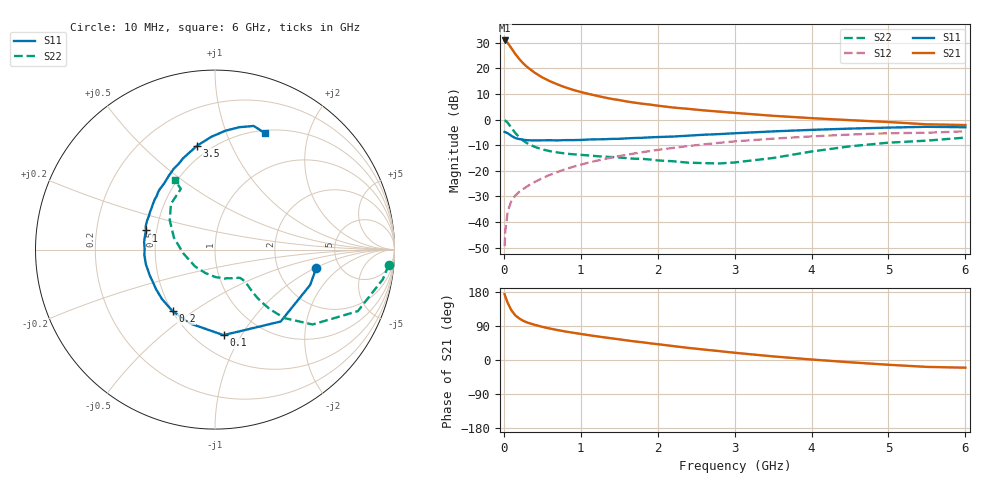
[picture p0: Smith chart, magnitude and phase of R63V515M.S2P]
! SIEMENS Small Signal Semiconductors
! BFR193
! Si NPN RF Bipolar Junction Transistor in SOT23
! VCE = 3.5 V  IC = 15 mA
! Common Emitter S-Parameters:  May  1996
# GHz  S  MA  R  50
!  f  S11  S21  S12  S22
! GHz  MAG  ANG  MAG  ANG  MAG  ANG  MAG  ANG
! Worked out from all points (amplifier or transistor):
!   36 points, 10 MHz to 6 GHz, reference 50 ohm
!   highest |S21| = 30.8 dB at 10 MHz (marker M1)
!   |S21| within 3 dB of that: start of sweep to 97.87 MHz
!   unconditionally stable (mu >= 1): 636.5 MHz to 1.893 GHz
!   at 250 MHz: K = 0.76, MSG = 24.5 dB, |S12| = -27.1 dB
!   at 1.4 GHz: K = 1.03, MAG = 10.4 dB, |S12| = -14.8 dB
!   at 6 GHz: K = 0.95, MSG = 1.2 dB, |S12| = -4.6 dB
!   S11 on the Smith chart (normalised r, x): 10 MHz: 3.34, -1.03; 100 MHz: 0.68, -0.84; 200 MHz: 0.50, -0.42; 1 GHz: 0.44, +0.11; 3.5 GHz: 0.42, +0.75; 6 GHz: 0.53, +1.38
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0.01  0.5732 -10.4  34.77 173.6  0.0034 87.1  0.9721 -5.0
0.02  0.5656 -20.4  34.42 167.2  0.0069 81.4  0.9498 -10.0
0.05  0.5426 -47.6  31.15 150.8  0.0159 70.2  0.8667 -23.3
0.1  0.4788 -84.3  24.36 130.7  0.0266 63.3  0.6854 -37.5
0.15  0.4346 -108.5  18.84 117.7  0.0331 59.7  0.5436 -44.6
0.2  0.4165 -124.6  15.17 109.7  0.0389 59.7  0.4538 -47.3
0.25  0.404 -137.0  12.52 103.6  0.0441 60.3  0.3898 -48.5
0.3  0.3957 -145.8  10.66 99.2  0.0495 62.1  0.3468 -48.7
0.4  0.3908 -158.5  8.206 92.9  0.0605 64.0  0.2939 -48.1
0.5  0.3936 -167.9  6.617 87.5  0.0718 65.1  0.2619 -47.2
0.6  0.3948 -175.3  5.578 82.9  0.0837 66.1  0.2413 -47.0
0.7  0.3923 179.1  4.823 78.9  0.0954 66.5  0.2282 -47.3
0.8  0.3973 173.7  4.237 75.2  0.1076 66.6  0.2175 -48.0
1  0.4 164.5  3.437 68.8  0.1317 65.8  0.2048 -50.0
1.1  0.4074 161.2  3.163 65.7  0.1441 65.1  0.1997 -52.2
1.3  0.4128 153.4  2.707 59.9  0.169 63.5  0.1886 -56.2
1.6  0.4297 143.4  2.244 51.6  0.2062 60.6  0.1765 -64.9
2.2  0.4657 127.3  1.714 36.8  0.2799 53.4  0.1537 -88.5
3.5  0.5872 99.8  1.182 9.5  0.4238 34.3  0.1779 -173.3
4.5  0.6654 84.9  0.972 -6.0  0.5094 19.8  0.3003 147.1
5.5  0.7219 72.6  0.806 -18.2  0.5523 5.0  0.388 119.4
6  0.7061 66.9  0.781 -20.3  0.5898 0.7  0.4447 119.9
